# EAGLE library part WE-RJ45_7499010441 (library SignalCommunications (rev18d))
WE-RJ45 LAN THT Surge Protection Characteristics: With two integrated gas discharge tubes High surge withstand voltage Small capacitance of surge device Application: Telecom devices Bridges, hubs, router, power line adapter LAN networks in rough environments Details see: http://katalog.we-online.de/en/pbs/WE-LAN_RJ45/7499010441? Updated by Yingchun Shan 2016-08-26 2016(C) Würth Elektronik
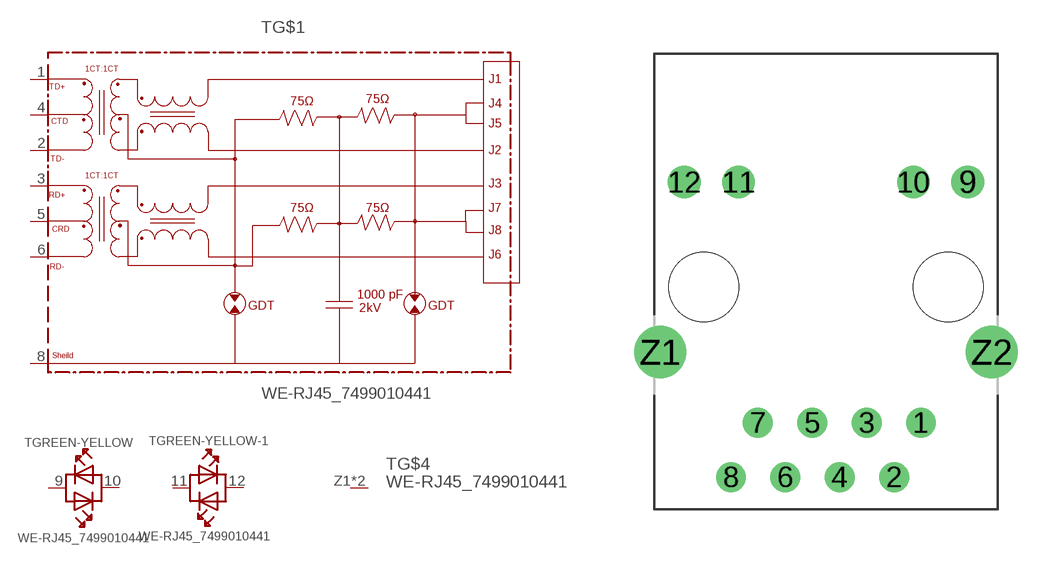
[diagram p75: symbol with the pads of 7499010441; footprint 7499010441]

Designator prefix T; gates G$1=7499010441 G$4=GNDPIN GREEN-YELLOW=LED-DUAL-1 GREEN-YELLOW-1=LED_DOUB-1

## WE-RJ45_7499010441  [7499010441]
1  G$1:TD+
2  G$1:TD-
3  G$1:RD+
4  G$1:CTD
5  G$1:CRD
6  G$1:RD-
8  G$1:SHIELD
9  GREEN-YELLOW:AK1  pas
10  GREEN-YELLOW:AK2  pas
11  GREEN-YELLOW-1:AK1  pas
12  GREEN-YELLOW-1:AK2  pas
Z1  G$4:GND  pwr
Z2  G$4:GND  pwr

## Footprint 7499010441 (pad centres in mm)
drill 0.89: 1 4.44,-6.35; 2 3.18,-8.89; 3 1.9,-6.35; 4 0.64,-8.89; 5 -0.64,-6.35; 6 -1.9,-8.89; 7 -3.18,-6.35; 8 -4.44,-8.89
drill 1.02: 9 6.625,4.9; 10 4.085,4.9; 11 -4.085,4.9; 12 -6.625,4.9
drill 1.63: Z1 -7.745,-3.05; Z2 7.745,-3.05
hole 3.25 at 5.715,0
hole 3.25 at -5.715,0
